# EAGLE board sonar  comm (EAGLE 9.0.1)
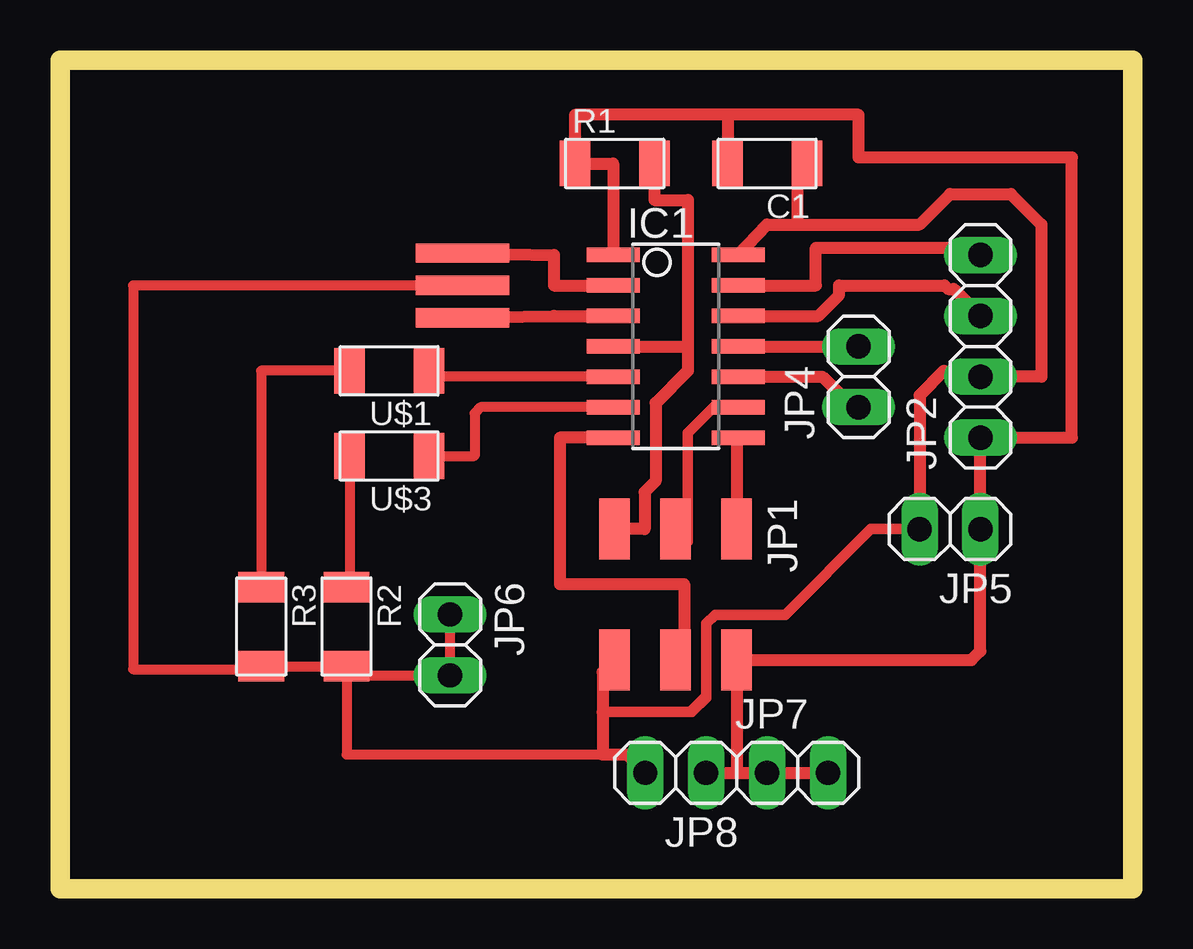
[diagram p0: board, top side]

Size 44.7 x 34.54 mm. Coordinates in mm from the lower left corner, seen from the top.
Outline: 0,34.54 0,0 44.7,0 44.7,34.54 0,34.54
Copper layers (1*16): Top 0.035mm / dielectric 1.5mm / Bottom 0.035mm
Design rules "default *": minimum track width 17mil, minimum drill 0.38mm, track to track 18mil, track to pad 16mil, pad to pad 16mil, via to via 16mil, smd to smd 16mil, copper to edge 40mil, drill to drill 6mil, minimum pad ring 10mil, minimum via ring 8mil, stop-mask expansion 4mil, vias tented up to drill 0mil, thermal gap 10mil

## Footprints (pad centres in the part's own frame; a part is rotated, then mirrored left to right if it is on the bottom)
C1206FAB = smd 1.27 x 1.905: 1 -1.651,0; 2 1.651,0
SOIC14 = smd 0.61 x 2.21: 1 -3.81,-2.603; 2 -2.54,-2.603; 3 -1.27,-2.603; 4 0,-2.603; 5 1.27,-2.603; 6 2.54,-2.603; 7 3.81,-2.603; 8 3.81,2.603; 9 2.54,2.603; 10 1.27,2.603; 11 0,2.603; 12 -1.27,2.603; 13 -2.54,2.603; 14 -3.81,2.603
2X03SMD = smd 2.54 x 1.27: 1 -2.54,2.54; 2 2.92,2.54; 3 -2.54,0; 4 2.92,0; 5 -2.54,-2.54; 6 2.92,-2.54
1X04 = drill 1.016 long: 1 -3.81,0; 2 -1.27,0; 3 1.27,0; 4 3.81,0
1X02 = drill 1.016 long: 1 -1.27,0; 2 1.27,0
R1206FAB = smd 1.27 x 1.905: 1 -1.651,0; 2 1.651,0
LED1206FAB = smd 1.27 x 1.905: 1 -1.651,0; 2 1.651,0
EFOBM = smd 0.8 x 3.9: 1 -1.35,0; 2 0,0; 3 1.35,0

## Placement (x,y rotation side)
C1  10uf  [C1206FAB]  29.46,30.23 180 top
IC1  ATTINY44-SSU  [SOIC14]  25.65,22.61 270 top
JP1  [2X03SMD]  25.65,12.45 270 top
JP2  [1X04]  38.35,22.61 90 top
JP4  [1X02]  33.27,21.34 90 top
JP5  [1X02]  37.08,14.99 180 top
JP6  [1X02]  16.26,10.16 270 top
JP7  [1X02]  30.73,4.83 0 top
JP8  [1X02]  25.65,4.83 180 top
R1  10k  [R1206FAB]  23.11,30.23 0 top
R2  [R1206FAB]  11.94,10.92 270 top
R3  [R1206FAB]  8.38,10.92 270 top
U$1  LEDFAB1206  [LED1206FAB]  13.72,21.59 180 top
U$2  RESONATOR  [EFOBM]  16.76,25.15 270 top
U$3  LEDFAB1206  [LED1206FAB]  13.72,18.03 180 top

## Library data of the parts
C1 IC1 JP1 R1-R3 U$1-U$3 = fab
JP2 JP4-JP8 = pinhead

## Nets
5V: C1.2 IC1.1 JP1.2 JP2.1 JP5.1 JP7.1 JP7.2 JP8.1 R1.1
GND: C1.1 IC1.14 JP1.6 JP2.2 JP5.2 JP6.1 JP6.2 JP8.2 R2.2 R3.2 U$2.2
N$3: IC1.11 JP4.2
N$4: IC1.7 JP1.4
N$5: IC1.4 JP1.5 R1.2
N$6: IC1.9 JP1.3
N$7: IC1.8 JP1.1
N$8: IC1.12 JP2.3
N$9: IC1.13 JP2.4
N$10: IC1.10 JP4.1
N$11: IC1.6 U$3.1
N$12: IC1.5 U$1.1
N$13: R3.1 U$1.2
N$14: R2.1 U$3.2
XTAL1: IC1.2 U$2.1
XTAL2: IC1.3 U$2.3

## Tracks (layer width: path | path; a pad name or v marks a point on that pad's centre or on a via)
5V
  Top 0.508: JP7.2 JP7.1 28.19,4.83 | JP8.1 28.19,4.83 | 28.19,4.83 JP1.2 37.97,9.53 38.35,9.91 JP5.1 JP2.1 42.16,18.8 42.16,30.48 33.27,30.48 33.27,32.26 27.81,32.26 | IC1.1 23.05,30.23 R1.1 21.46,32.26 27.81,32.26 | 27.81,32.26 C1.2
GND
  Top 0.406: R2.2 R3.2 8.26,9.14 3.05,9.14 3.05,25.15 U$2.2 15.49,25.15 | R2.2 11.94,5.59 22.61,5.59 | R2.2 12.32,8.89 JP6.2 JP6.1
  Top 0.432: 26.92,7.96 26.33,7.37 | 22.61,7.37 26.33,7.37 | JP5.2 33.78,14.99 30.21,11.42 27.3,11.42 26.94,11.05 26.94,8.02 26.33,7.42 26.33,7.37
  Top 0.508: IC1.14 29.46,27.69 30.73,27.69 | 30.73,27.69 30.73,30.23 C1.1 | 30.73,27.69 35.81,27.69 37.08,28.96 39.62,28.96 40.89,27.69 40.89,21.34 JP2.2 37.08,21.34 36.83,21.59 35.81,20.57 JP5.2 | JP1.6 22.61,9.02 22.61,7.37 22.61,5.59 23.62,5.59 JP8.2
N$3
  Top 0.508: IC1.11 JP4.2
N$4
  Top 0.508: IC1.7 20.83,18.8 20.83,12.7 26.01,12.7 26.01,9.53 JP1.4
N$5
  Top 0.508: R1.2 24.77,28.7 26.16,28.7 26.16,22.61 | 26.16,22.61 26.16,21.59 24.82,20.24 24.82,16.99 24.36,16.53 24.36,14.99 JP1.5 | IC1.4 26.16,22.61
N$6
  Top 0.432: JP1.3 26.16,14.48 26.16,18.99 27.24,20.07 IC1.9
N$7
  Top 0.508: IC1.8 28.19,18.73 JP1.1
N$8
  Top 0.508: IC1.12 31.59,23.88 32.46,24.75 32.46,25.15 36.85,25.15 37,24.99 37.24,24.99 JP2.3
N$9
  Top 0.508: JP2.4 38.35,26.72 31.5,26.72 31.5,25.15 IC1.13
N$10
  Top 0.508: IC1.10 31.75,21.34 33.27,19.81 JP4.1
N$11
  Top 0.406: U$3.1 17.27,18.03 17.27,19.81 17.53,20.07 IC1.6
N$12
  Top 0.406: IC1.5 15.62,21.34 U$1.1
N$13
  Top 0.406: U$1.2 8.38,21.59 R3.1
N$14
  Top 0.406: U$3.2 12.06,12.7 R2.1
XTAL1
  Top 0.508: U$2.1 20.57,26.42 20.57,25.15 IC1.2 23.11,25.15
XTAL2
  Top 0.508: U$2.3 20.57,23.88 IC1.3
